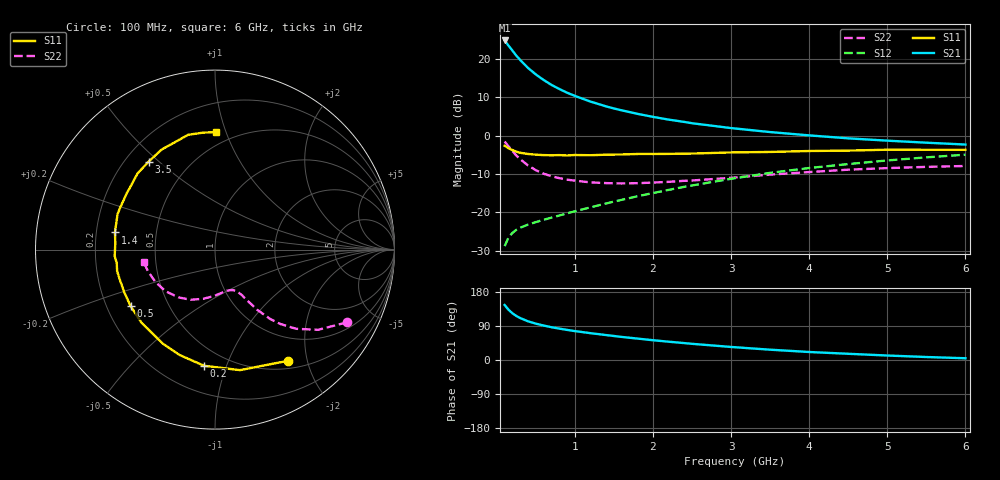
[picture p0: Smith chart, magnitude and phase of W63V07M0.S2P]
! SIEMENS Small Signal Semiconductors
! BFR193W
! Si NPN RF Bipolar Junction Transistor in SOT323
! VCE = 3 V  IC = 7 mA
! Common Emitter S-Parameters:  September  1992
# GHz  S  MA  R  50
!  f  S11  S21  S12  S22
! GHz  MAG  ANG  MAG  ANG  MAG  ANG  MAG  ANG
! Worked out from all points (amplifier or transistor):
!   28 points, 100 MHz to 6 GHz, reference 50 ohm
!   highest |S21| = 24.9 dB at 100 MHz (marker M1)
!   |S21| within 3 dB of that: start of sweep to 213.3 MHz
!   unconditionally stable (mu >= 1): 1.107 GHz to 2.565 GHz
!   at 300 MHz: K = 0.45, MSG = 21.9 dB, |S12| = -24.0 dB
!   at 1.5 GHz: K = 1.06, MAG = 10.7 dB, |S12| = -17.2 dB
!   at 6 GHz: K = 0.90, MSG = 1.3 dB, |S12| = -4.9 dB
!   lowest NFmin = 1.20 dB at 450 MHz
!   S11 on the Smith chart (normalised r, x): 100 MHz: 0.61, -1.68; 200 MHz: 0.37, -0.84; 500 MHz: 0.30, -0.28; 1.4 GHz: 0.28, +0.08; 3.5 GHz: 0.29, +0.46; 6 GHz: 0.40, +0.92
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0.1  0.7406 -56.8  17.5 145.2  0.0362 63.4  0.8406 -28.8
0.15  0.6858 -78.3  15 132.7  0.047 55.8  0.7275 -37.9
0.2  0.6501 -95.4  12.89 123.3  0.054 50.5  0.6318 -44.3
0.25  0.6191 -108.8  11.11 116.2  0.0592 47.5  0.5516 -48.7
0.3  0.599 -119.1  9.714 110.6  0.0631 45.7  0.4942 -51.5
0.4  0.5776 -135.2  7.661 102.1  0.0692 44.8  0.4086 -55.0
0.5  0.5658 -146.3  6.299 95.9  0.0746 45.5  0.3551 -56.8
0.6  0.5587 -155.0  5.335 90.9  0.08 46.9  0.3191 -58.4
0.7  0.5559 -161.8  4.604 86.5  0.0853 48.7  0.2959 -59.3
0.8  0.5585 -167.5  4.073 82.8  0.0909 50.4  0.2795 -60.7
0.9  0.5526 -172.2  3.639 79.4  0.0971 52.2  0.2671 -61.6
1  0.5601 -176.3  3.309 76.3  0.1033 53.7  0.2592 -63.1
1.2  0.5567 176.3  2.788 70.8  0.1163 56.3  0.2461 -66.4
1.4  0.5655 170.3  2.414 65.8  0.1306 58.4  0.2409 -69.8
1.8  0.5778 160.1  1.931 56.5  0.1621 61.2  0.2401 -78.0
2.2  0.5792 151.1  1.623 48.3  0.1964 62.3  0.2501 -86.2
2.5  0.585 145.0  1.455 42.7  0.2244 62.1  0.2604 -92.5
3  0.6051 135.5  1.258 34.4  0.2739 60.6  0.2823 -103.7
3.5  0.614 127.0  1.116 27.2  0.3276 57.7  0.3109 -116.0
4.5  0.6392 110.1  0.924 16.4  0.4267 49.3  0.3604 -140.0
5.5  0.6549 96.0  0.811 7.9  0.5219 40.0  0.3922 -161.9
6  0.6548 89.7  0.767 4.6  0.5656 34.7  0.4029 -169.9
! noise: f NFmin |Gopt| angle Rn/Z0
0.45  1.2  0.24  125  0.12
0.9  1.25  0.36  154  0.11
1.8  2  0.55  -156  0.13
